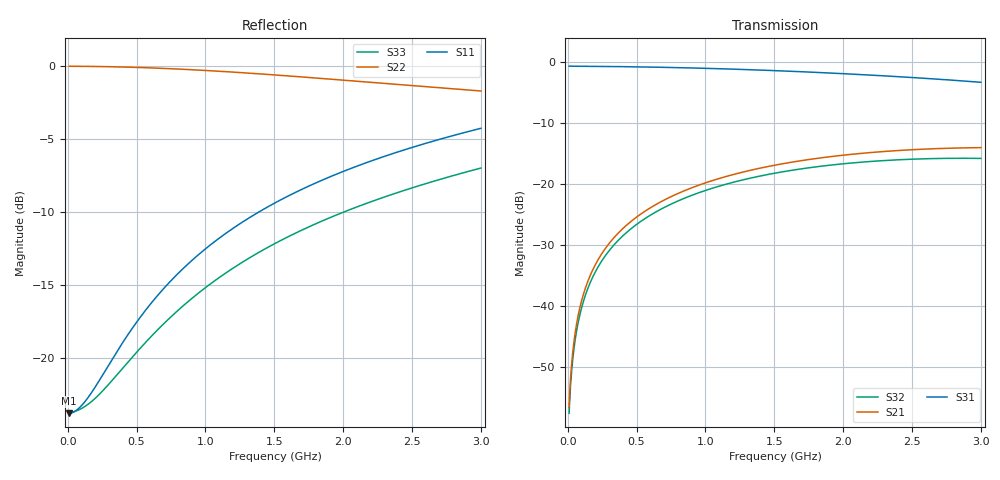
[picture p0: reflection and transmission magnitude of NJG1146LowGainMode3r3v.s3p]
! Created Mon Oct 18 18:45:01 2010
# hz S ma R 50
! 3 Port Network Data Port1:RFIN  Port2:RFOUT1  Port3:RFOUT2
! freq  magS11  angS11  magS12  angS12  magS13  angS13
!  magS21  angS21
!  magS22  angS22  magS23  angS23
!  magS31  angS31  magS32  angS32
!  magS33  angS33
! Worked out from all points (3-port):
!   2991 points, 10 MHz to 3 GHz, reference 50 ohm
!   strongest paths, dB at 10 MHz, 757 MHz, 1.505 GHz, 2.253 GHz, 3 GHz:
!     S31: -0.6, -0.8, -1.3, -2.1, -3.3
!     S21: -56.5, -22.0, -16.9, -14.7, -14.0
!     S32: -57.6, -23.2, -18.2, -16.2, -15.8
!   lowest |S11| = -23.8 dB at 10 MHz (marker M1), VSWR 1.14, Z = 56.9 - j0.313 ohm
!   |S11| at or under -10 dB: start of sweep to 1.389 GHz
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1e7  0.06465 -2.4  0.001478 69.7  0.932 -0.2
     0.001488 70.2  0.9968 -0.4  0.001327 69.9
     0.932 -0.2  0.001319 69.5  0.06506 -1.9
5.1e7  0.06563 -12.1  0.005633 80.6  0.9315 -1.2
       0.005721 80.9  0.9959 -1.4  0.005087 80.8
       0.9315 -1.2  0.00501 80.6  0.0656 -9.2
1.08e8  0.06935 -24.5  0.01168 82.5  0.9307 -2.4
        0.01187 82.6  0.9956 -3.0  0.01055 82.7
        0.9307 -2.4  0.01038 82.6  0.06747 -19.0
2.01e8  0.07974 -41.5  0.02159 80.9  0.9289 -4.5
        0.02195 81.0  0.9944 -5.6  0.01948 81.1
        0.9289 -4.5  0.01916 81.1  0.07286 -33.4
3.36e8  0.1013 -59.0  0.03589 76.9  0.9255 -7.4
        0.03649 77.0  0.9919 -9.3  0.03234 77.2
        0.9255 -7.4  0.03181 77.2  0.08522 -50.3
5.32e8  0.139 -75.3  0.05619 70.5  0.919 -11.6
        0.05713 70.5  0.9861 -14.6  0.05056 71.0
        0.919 -11.6  0.04972 70.9  0.1087 -68.2
7.89e8  0.1921 -89.2  0.08158 61.8  0.9073 -17.2
        0.08296 61.8  0.9752 -21.5  0.07324 62.5
        0.9073 -17.2  0.07203 62.5  0.1439 -84.4
1.505e9  0.3394 -114.0  0.1412 37.9  0.8567 -32.2
         0.1436 37.9  0.9302 -40.1  0.1256 39.2
         0.8567 -32.2  0.1234 39.2  0.2465 -113.5
2.219e9  0.4751 -132.4  0.1798 14.9  0.7851 -46.9
         0.183 15.0  0.8761 -57.5  0.1572 16.9
         0.7851 -46.9  0.1545 16.9  0.3448 -134.9
3e9  0.6109 -150.2  0.1963 -9.2  0.6874 -62.9
     0.1999 -9.2  0.8198 -75.6  0.1661 -6.3
     0.6874 -62.9  0.1631 -6.3  0.4465 -155.5
